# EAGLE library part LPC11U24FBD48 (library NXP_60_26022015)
32-bit ARM Cortex-M0 microcontroller; up to 32 kB flash; up to 10 kB SRAM and 4 kB EEPROM; USB device; USART The LPC11U2x are an ARM Cortex-M0 based, low-cost 32-bit MCU family, designed for 8/16-bit microcontroller applications, offering performance, low power, simple instruction set and memory addressing together with reduced code size compared to existing 8/16-bit architectures. The LPC11U2x operate at CPU frequencies of up to 50 MHz. Equipped with a highly flexible and configurable Full-Speed USB 2.0 device controller, the LPC11U2x brings unparalleled design flexibility and seamless integration to today’s demanding connectivity solutions. The peripheral complement of the LPC11U2x includes up to 32 kB of flash memory, up to 10 kB of SRAM data memory and 4 kB EEPROM, one Fast-mode Plus I 2 C-bus interface, one RS-485/EIA-485 USART with support for synchronous mode and smart card interface, two SSP interfaces, four general-purpose counter/timers, a 10-bit ADC (Analog-to-Digital Converter), and up to 54 general-purpose I/O pins. AAL Eindhoven MK
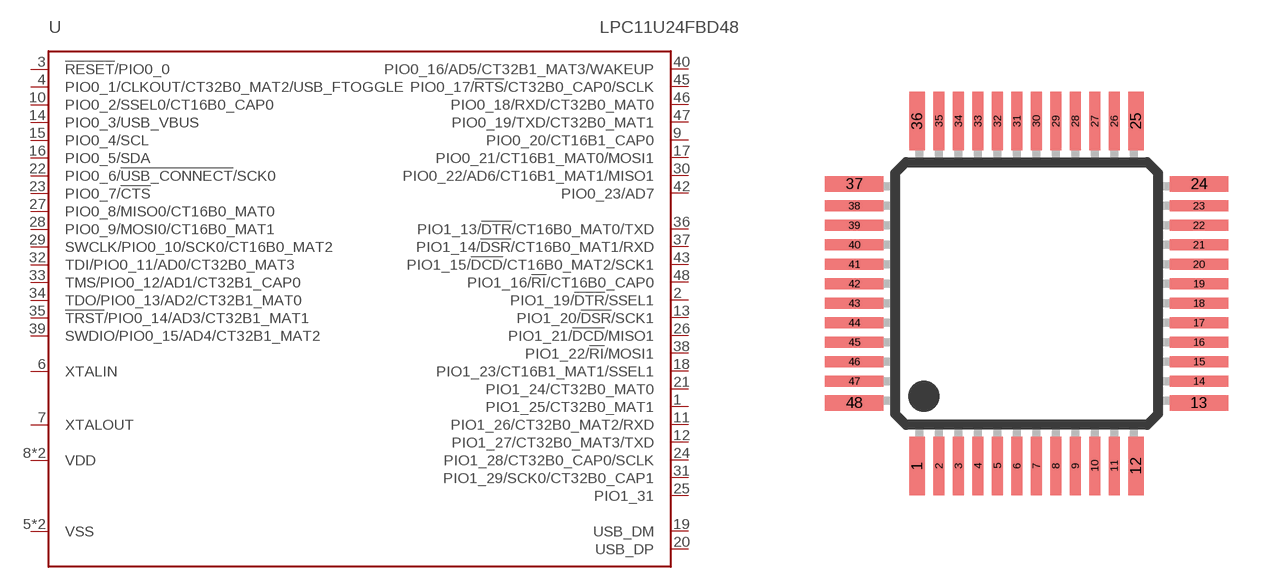
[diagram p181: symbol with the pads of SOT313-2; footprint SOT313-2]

Designator prefix U

## LPC11U24FBD48/301 (EEPROM: 2kB; FLASH: 32kB; GPIO: 40; SRAM: 6kB; USB_SRAM: 2kB), LPC11U24FBD48/401 (EEPROM: 4kB; FLASH: 32kB; GPIO: 40; SRAM: 8kB; USB_SRAM: 2kB)  [SOT313-2]
1  PIO1_25/CT32B0_MAT1
2  PIO1_19/!DTR!/SSEL1
3  !RESET!/PIO0_0
4  PIO0_1/CLKOUT/CT32B0_MAT2/USB_FTOGGLE
5  VSS  pwr
6  XTALIN  in
7  XTALOUT  out
8  VDD  pwr
9  PIO0_20/CT16B1_CAP0
10  PIO0_2/SSEL0/CT16B0_CAP0
11  PIO1_26/CT32B0_MAT2/RXD
12  PIO1_27/CT32B0_MAT3/TXD
13  PIO1_20/!DSR!/SCK1
14  PIO0_3/USB_VBUS
15  PIO0_4/SCL
16  PIO0_5/SDA
17  PIO0_21/CT16B1_MAT0/MOSI1
18  PIO1_23/CT16B1_MAT1/SSEL1
19  USB_DM
20  USB_DP
21  PIO1_24/CT32B0_MAT0
22  PIO0_6/!USB_CONNECT!/SCK0
23  PIO0_7/!CTS!
24  PIO1_28/CT32B0_CAP0/SCLK
25  PIO1_31
26  PIO1_21/!DCD!/MISO1
27  PIO0_8/MISO0/CT16B0_MAT0
28  PIO0_9/MOSI0/CT16B0_MAT1
29  SWCLK/PIO0_10/SCK0/CT16B0_MAT2
30  PIO0_22/AD6/CT16B1_MAT1/MISO1
31  PIO1_29/SCK0/CT32B0_CAP1
32  TDI/PIO0_11/AD0/CT32B0_MAT3
33  TMS/PIO0_12/AD1/CT32B1_CAP0
34  TDO/PIO0_13/AD2/CT32B1_MAT0
35  !TRST!/PIO0_14/AD3/CT32B1_MAT1
36  PIO1_13/!DTR!/CT16B0_MAT0/TXD
37  PIO1_14/!DSR!/CT16B0_MAT1/RXD
38  PIO1_22/!RI!/MOSI1
39  SWDIO/PIO0_15/AD4/CT32B1_MAT2
40  PIO0_16/AD5/CT32B1_MAT3/WAKEUP
41  VSS  pwr
42  PIO0_23/AD7
43  PIO1_15/!DCD!/CT16B0_MAT2/SCK1
44  VDD  pwr
45  PIO0_17/!RTS!/CT32B0_CAP0/SCLK
46  PIO0_18/RXD/CT32B0_MAT0
47  PIO0_19/TXD/CT32B0_MAT1
48  PIO1_16/!RI!/CT16B0_CAP0

## Footprint SOT313-2 (pad centres in mm)
SOT313-2 LQFP48: plastic low profile quad flat package; 48 leads; body 7 x 7 x 1.4 mm JEDEC: MS-026 IEC: 136E05 Footprint according to NXP SOT313-2 specification, however the cornerpins are 0.4mm in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
smd 0.4 x 1.5: 1 -2.81,-4.425; 12 2.81,-4.425; 25 2.81,4.425; 36 -2.81,4.425
smd 0.28 x 1.5: 2 -2.25,-4.425; 3 -1.75,-4.425; 4 -1.25,-4.425; 5 -0.75,-4.425; 6 -0.25,-4.425; 7 0.25,-4.425; 8 0.75,-4.425; 9 1.25,-4.425; 10 1.75,-4.425; 11 2.25,-4.425; 26 2.25,4.425; 27 1.75,4.425; 28 1.25,4.425; 29 0.75,4.425; 30 0.25,4.425; 31 -0.25,4.425; 32 -0.75,4.425; 33 -1.25,4.425; 34 -1.75,4.425; 35 -2.25,4.425
smd 1.5 x 0.4: 13 4.425,-2.81; 24 4.425,2.81; 37 -4.425,2.81; 48 -4.425,-2.81
smd 1.5 x 0.28: 14 4.425,-2.25; 15 4.425,-1.75; 16 4.425,-1.25; 17 4.425,-0.75; 18 4.425,-0.25; 19 4.425,0.25; 20 4.425,0.75; 21 4.425,1.25; 22 4.425,1.75; 23 4.425,2.25; 38 -4.425,2.25; 39 -4.425,1.75; 40 -4.425,1.25; 41 -4.425,0.75; 42 -4.425,0.25; 43 -4.425,-0.25; 44 -4.425,-0.75; 45 -4.425,-1.25; 46 -4.425,-1.75; 47 -4.425,-2.25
